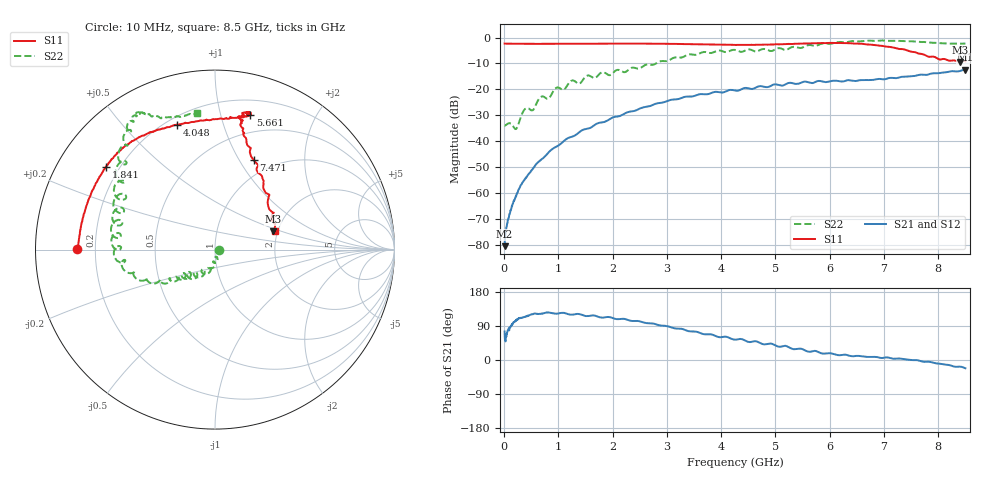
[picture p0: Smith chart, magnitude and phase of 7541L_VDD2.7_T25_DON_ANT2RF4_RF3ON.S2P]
!Agilent Technologies,E5071C,MY46417908,A.11.23
!Date: Wed Dec 09 17:18:09 2020
!Data & Calibration Information:
!Freq	S11:SOLT2(ON)	S21:SOLT2(ON)	S12:SOLT2(ON)	S22:SOLT2(ON)
!PortZ  Port1:50+j0  Port2:50+j0
!Above PortZ is port z conversion or system Z0 setting when saving the data.
!When reading, reference impedance value at option line is always used.
# Hz S dB R 50
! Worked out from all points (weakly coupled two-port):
!   1601 points, 10 MHz to 8.5 GHz, reference 50 ohm
!   highest |S21| = -12.44 dB at 8.5 GHz (marker M1); lowest = -80.5 dB at 10 MHz (marker M2)
!   lowest |S11| = -9.4 dB at 8.41 GHz (marker M3), VSWR 2.02, Z = 94.3 + j21.8 ohm
!   |S11| at or under -10 dB: nowhere
!   |S22| runs from -35.3 to -1.1 dB; largest |S21 - S12| = 0.0031
!   S11 on the Smith chart (normalised r, x): 10 MHz: 0.13, +0.00; 1.841 GHz: 0.15, +0.33; 4.048 GHz: 0.24, +0.71; 5.661 GHz: 0.33, +1.24; 7.471 GHz: 0.81, +1.15; 8.5 GHz: 1.92, +0.46
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1e7  -2.30 179.7  -80.49 75.1  -79.01 54.2  -33.89 -5.7
1.002062e8  -2.36 177.9  -68.28 85.5  -68.16 82.0  -32.99 -42.7
2.2225e8  -2.39 175.2  -61.23 105.1  -61.01 104.6  -35.30 -54.9
3.761312e8  -2.39 172.1  -54.94 113.6  -54.84 113.5  -27.75 -68.0
5.247062e8  -2.41 169.0  -50.77 120.6  -50.60 120.1  -28.05 -82.5
6.732812e8  -2.42 166.0  -47.27 121.9  -47.28 121.9  -22.97 -86.7
8.643062e8  -2.42 161.9  -43.41 124.3  -43.42 124.3  -22.31 -89.8
1.24105e9  -2.39 154.4  -38.31 119.6  -38.35 119.5  -16.66 -111.7
1.426769e9  -2.38 150.9  -35.88 119.8  -35.90 119.6  -17.09 -114.1
1.840656e9  -2.35 142.8  -32.61 112.0  -32.61 112.0  -13.43 -136.1
2.843538e9  -2.37 128.0  -25.29 92.2  -25.30 92.3  -9.44 -145.8
3.612944e9  -2.60 116.4  -21.83 71.2  -21.84 71.2  -6.03 -165.0
4.048056e9  -2.75 107.0  -21.09 61.4  -21.10 61.3  -5.46 177.8
4.255e9  -2.84 102.0  -20.41 53.7  -20.41 53.7  -4.77 173.3
5.236656e9  -2.45 79.5  -17.53 34.5  -17.52 34.5  -4.39 152.3
5.661156e9  -2.22 75.3  -17.56 22.2  -17.50 22.2  -2.94 136.2
5.671769e9  -2.20 75.4  -17.57 22.6  -17.51 22.6  -2.98 135.8
6.446481e9  -2.33 78.0  -16.75 10.0  -16.76 10.2  -1.34 123.3
7.088538e9  -3.52 76.3  -15.61 6.2  -15.67 6.1  -1.26 118.9
7.470588e9  -5.27 66.8  -14.97 0.6  -14.97 0.5  -1.44 117.0
8.409794e9  -9.42 17.6  -12.81 -17.5  -12.86 -17.7  -2.33 99.4
8.5e9  -9.17 17.5  -12.44 -21.8  -12.53 -21.6  -2.29 97.4
